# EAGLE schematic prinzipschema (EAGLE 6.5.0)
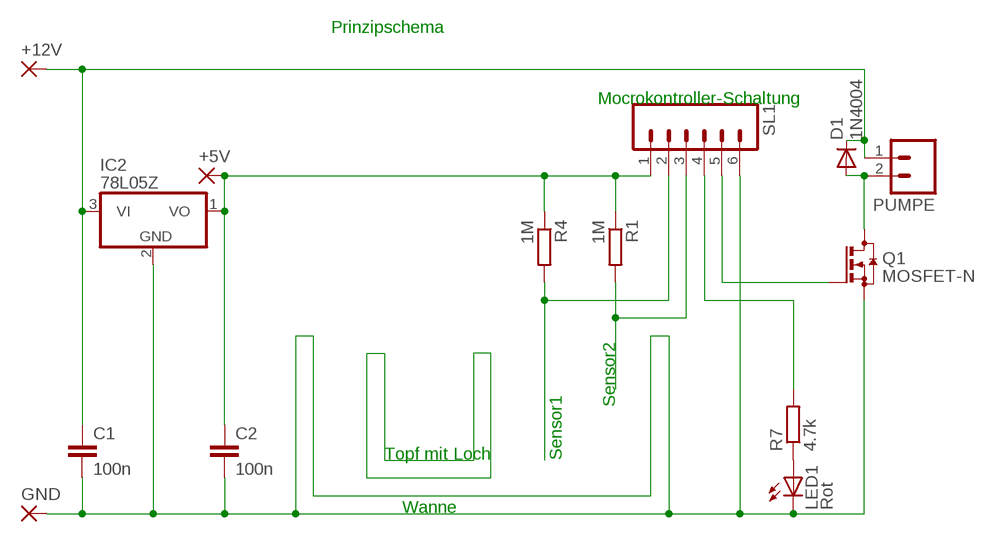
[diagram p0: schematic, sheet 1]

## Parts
+5V  2,54/1,0  [2,54/1,0]
+12V  2,54/1,0  [2,54/1,0]
C1  100n  C2,5-3  [C2.5-3]
C2  100n  C2,5-3  [C2.5-3]
D1  1N4004  [DO41-10]
GND  2,54/1,0  [2,54/1,0]
IC2  78L05Z  [TO92]
LED1  Rot  TLLG4400  [LED3MM]
PUMPE  M02  [02P]
Q1  MOSFET-N  BSS123  [SOT23]
R1  1M  R-EU_M1206  [M1206]
R4  1M  R-EU_M1206  [M1206]
R7  4.7k  R-EU_R0805  [R0805]
SL1  M06  [06P]

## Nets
GND [dick2]: C1.2 C2.2 GND.1(P) IC2.2(GND) LED1.K(C) Q1.2(S) SL1.6
N$1: R4.2 SL1.2
N$2: +12V.1(P) C1.1 D1.C IC2.3(VI) PUMPE.1
N$3: R1.2 SL1.3
N$5: R7.2 SL1.4
N$6: D1.A PUMPE.2 Q1.3(D)
N$8: Q1.1(G) SL1.5
N$15: LED1.A R7.1
VCC [dick]: +5V.1(P) C2.1 IC2.1(VO) R1.1 R4.1 SL1.1

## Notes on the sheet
- Prinzipschema
- Mocrokontroller-Schaltung
- Sensor2
- Topf mit Loch | Sensor1
- Wanne

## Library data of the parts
+5V +12V GND = wirepad:2,54/1,0: THROUGH-HOLE PAD
C1 C2 = capacitor-wima:C: CAPACITOR
D1 = diode:1N4004: DIODE
IC2 = linear:78*: Positive VOLTAGE REGULATOR Source: http://cache.national.com/ds/LM/LM78L05.pdf http://www.fairchildsemi.com/ds/LM/LM7805.pdf
LED1 = led:TLLG4400: Low Current (2mA) LED 3 mm Tinted Diffused Package color GREEN; MF: VISHAY SEMICONDUCTOR; OC_FARNELL: 1612435
PUMPE = con-amp-quick:M02: AMP QUICK CONNECTOR; OC_FARNELL: unknown; OC_NEWARK: unknown
Q1 = transistor-small-signal:BSS123: N-CHANNEL MOS FET
R1 R4 R7 = rcl:R-EU_: RESISTOR, European symbol
SL1 = con-amp-quick:M06: AMP QUICK CONNECTOR; OC_FARNELL: unknown; OC_NEWARK: unknown

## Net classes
1 dick: width 0.762 mm
2 dick2: width 1.016 mm, drill 0.762 mm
